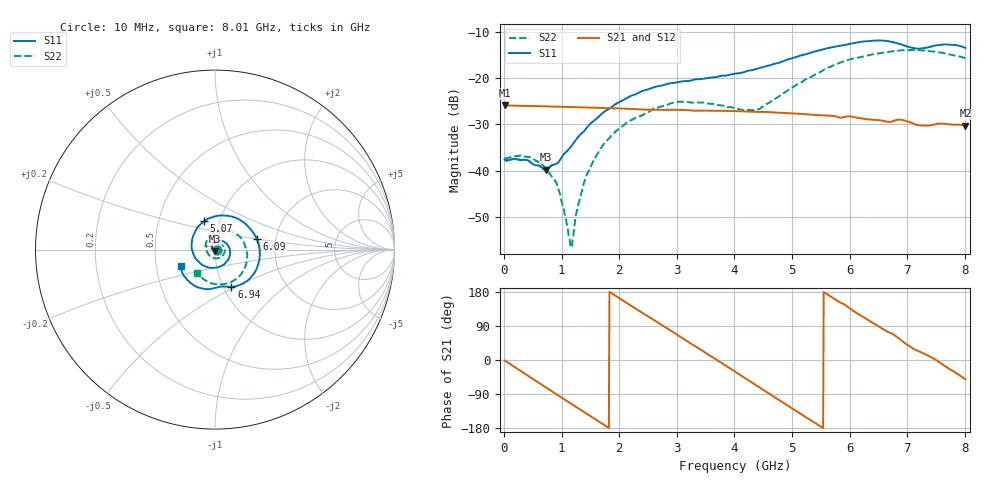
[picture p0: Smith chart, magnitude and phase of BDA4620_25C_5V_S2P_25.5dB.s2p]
!Agilent Technologies,E5071B,MY42404982,A.09.10
!Date: Wed May 06 09:03:58 2026
!Data & Calibration Information:
!Freq	S11:SOLT2(ON)	S21:SOLT2(ON)	S12:SOLT2(ON)	S22:SOLT2(ON)
# Hz S RI R 50
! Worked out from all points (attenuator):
!   801 points, 10 MHz to 8.01 GHz, reference 50 ohm
!   highest |S21| = -25.90 dB at 10 MHz (marker M1); lowest = -30.3 dB at 8.01 GHz (marker M2)
!   lowest |S11| = -39.8 dB at 720 MHz (marker M3), VSWR 1.02, Z = 49.7 - j0.993 ohm
!   |S11| at or under -10 dB: start of sweep to end of sweep
!   |S22| runs from -56.3 to -13.9 dB; largest |S21 - S12| = 0.00026
!   S11 on the Smith chart (normalised r, x): 10 MHz: 1.03, -0.00; 5.07 GHz: 0.84, +0.27; 6.09 GHz: 1.59, +0.20; 6.94 GHz: 1.09, -0.48; 8.01 GHz: 0.67, -0.13
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1e7  0.0132 -0.000836  0.0507 -0.00105  0.0508 -0.0011  0.0135 -0.000402
4.4e8  0.00814 -0.00975  0.036 -0.0347  0.036 -0.0348  0.0131 -0.0048
7.2e8  -0.00243 -0.00998  0.0156 -0.0471  0.0156 -0.0472  0.00839 -0.00689
9.4e8  -0.0114 -0.00465  -0.00285 -0.0491  -0.00288 -0.0492  0.00325 -0.0055
1.16e9  -0.017 0.00643  -0.0205 -0.0442  -0.0206 -0.0443  -0.0013 -0.000798
1.19e9  -0.0174 0.00829  -0.0227 -0.043  -0.0228 -0.0431  -0.00176 0.000127
1.27e9  -0.0179 0.0135  -0.0283 -0.0394  -0.0284 -0.0394  -0.00289 0.00233
1.35e9  -0.0173 0.0186  -0.0334 -0.035  -0.0334 -0.035  -0.00329 0.00488
1.53e9  -0.0124 0.0311  -0.042 -0.0232  -0.042 -0.0232  -0.00308 0.0115
1.77e9  0.00243 0.0444  -0.0473 -0.0046  -0.0474 -0.00463  0.00108 0.0205
2.15e9  0.0392 0.0478  -0.0398 0.0244  -0.0399 0.0244  0.0173 0.0291
2.68e9  0.0821 0.00392  -0.00634 0.0452  -0.0063 0.0452  0.0443 0.0192
3.08e9  0.0749 -0.0537  0.023 0.0389  0.0232 0.039  0.055 -0.00756
4.01e9  -0.0768 -0.081  0.0378 -0.0225  0.0379 -0.0226  -0.0107 -0.0464
4.43e9  -0.1285 0.00246  0.0136 -0.0409  0.0137 -0.041  -0.045 -0.0116
5.07e9  -0.0608 0.1577  -0.0289 -0.0296  -0.029 -0.0297  -0.0227 0.0812
5.35e9  0.0222 0.1896  -0.0381 -0.0128  -0.0382 -0.0128  0.0232 0.1023
6.09e9  0.2335 0.0588  -0.0226 0.0302  -0.0227 0.0303  0.1585 0.0436
6.68e9  0.1823 -0.1721  0.00974 0.0322  0.00971 0.0323  0.1699 -0.0902
6.94e9  0.0915 -0.207  0.0241 0.0254  0.0241 0.0255  0.1371 -0.1472
7.58e9  -0.0793 -0.2149  0.0319 -0.00471  0.032 -0.00467  -0.0178 -0.1881
8.01e9  -0.1919 -0.0907  0.0193 -0.0236  0.0194 -0.0237  -0.1029 -0.1282
